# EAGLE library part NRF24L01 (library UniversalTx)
nRF24L01 Single chip 2.4GHz transceiver from Nordic Semiconductors.
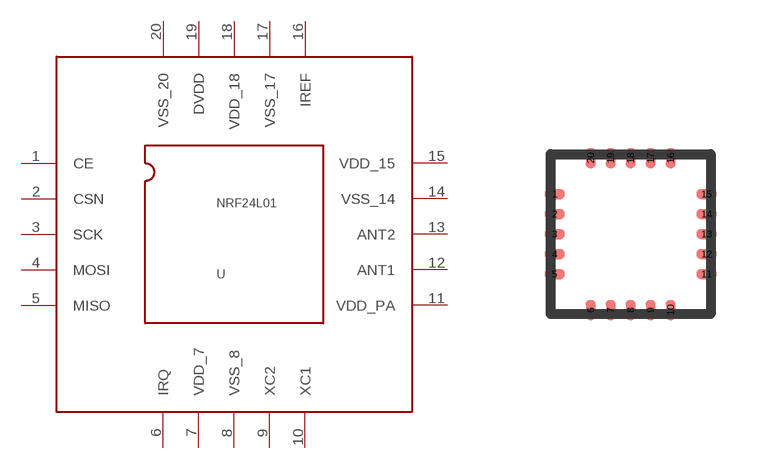
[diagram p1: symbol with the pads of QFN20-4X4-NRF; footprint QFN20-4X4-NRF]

Designator prefix -

## NRF24L01  [QFN20-4X4-NRF]
1  CE
2  CSN
3  SCK
4  MOSI
5  MISO
6  IRQ
7  VDD_7
8  VSS_8
9  XC2
10  XC1
11  VDD_PA
12  ANT1
13  ANT2
14  VSS_14
15  VDD_15
16  IREF
17  VSS_17
18  VDD_18
19  DVDD
20  VSS_20

## Footprint QFN20-4X4-NRF (pad centres in mm)
QFN20 4mm x 4mm package, with matt tin plating from Nordic Semiconductor.
smd 0.5 x 0.25: 1 -1.9,1; 2 -1.9,0.5; 3 -1.9,0; 4 -1.9,-0.5; 5 -1.9,-1; 11 1.9,-1; 12 1.9,-0.5; 13 1.9,0; 14 1.9,0.5; 15 1.9,1
smd 0.25 x 0.5: 6 -1,-1.9; 7 -0.5,-1.9; 8 0,-1.9; 9 0.5,-1.9; 10 1,-1.9; 16 1,1.9; 17 0.5,1.9; 18 0,1.9; 19 -0.5,1.9; 20 -1,1.9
